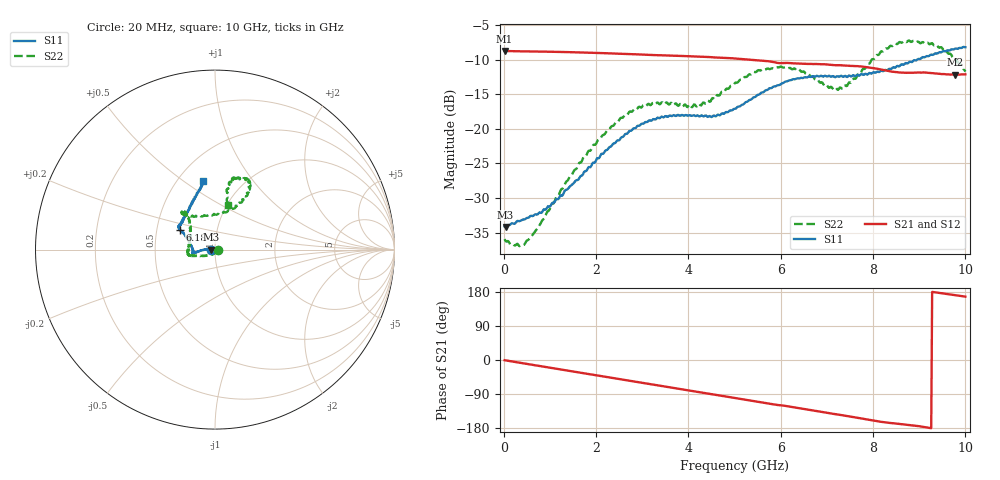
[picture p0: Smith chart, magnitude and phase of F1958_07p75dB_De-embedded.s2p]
! Integrated Device Technology
! Corporate Headquarters
! 6024 Silver Creek Valley Road
! San Jose, CA 95138  USA
! Phone:  1-408-284-8200
! Toll Free:  1-800-223-1366
! Webpage:  http://www.idt.com/
! Timing and RF Division
! 515 Groton Road, Suite 102
! Westford, MA 01886-6024
! Device:  F1958
! Description: 7-bit 0.25 dB Digital Step Attenuator
! Frequency:  0.001 -  6.000 GHz
! Package:  4x4 mm Thin QFN Plastic Package: 24 pin
! Ports:  2 RF, 12 DC
!  Pin  1  = D0
!  Pin  2  = VDD
!  Pin  3  = VMODE
!  Pin  4  = GND
!  Pin  5  = RF1  =  Port 1
!  Pin  6  = GND
!  Pin  7  = GND
!  Pin  8  = GND
!  Pin  9  = GND
!  Pin 10  = GND
!  Pin 11  = GND
!  Pin 12  = GND
!  Pin 13  = GND
!  Pin 14  = RF2  =  Port 2
!  Pin 15  = GND
!  Pin 16  = LE
!  Pin 17  = CLK
!  Pin 18  = DATA
!  Pin 19  = D6
!  Pin 20  = D5
!  Pin 21  = D4
!  Pin 22  = D3
!  Pin 23  = D2
!  Pin 24  = D1
! State:  31
! Atten State:  7.75 dB
! Voltage:  +3.30 Volts
! Current:  0.258 mA
! Data:  The device was measured on a F1958 evaluation board which has
!  individual transmission lines to the RF pins.  Data was collected
!  using a calibrated network analyzer.  The evaluation board was
!  de-embedded using Automatic Fixture Removal (AFR).
!  The reference plane is the edge of the package pin.
! Misc:
!  Action Tracker AT0419
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# GHz S dB R 50
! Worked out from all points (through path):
!   500 points, 20 MHz to 10 GHz, reference 50 ohm
!   highest |S21| = -8.75 dB at 20 MHz (marker M1); lowest = -12.2 dB at 9.78 GHz (marker M2)
!   group delay of S21, straight-line fit = 54.1 ps
!   lowest |S11| = -34.2 dB at 40 MHz (marker M3), VSWR 1.04, Z = 48.1 - j0.0778 ohm
!   |S11| at or under -10 dB: start of sweep to 8.959 GHz
!   |S22| runs from -37.0 to -7.2 dB; largest |S21 - S12| = 0.0011
!   S11 on the Smith chart (normalised r, x): 20 MHz: 0.96, -0.00; 6.18 GHz: 0.66, +0.15; 10 GHz: 0.66, +0.60
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0.02  -34.13 -177.6  -8.75 -0.6  -8.75 -0.5  -35.95 -8.9
0.04  -34.18 -177.6  -8.76 -1.0  -8.76 -0.9  -36.22 -13.5
0.46  -33.07 173.7  -8.82 -9.4  -8.82 -9.4  -36.60 -59.7
0.96  -31.20 175.4  -8.87 -19.5  -8.86 -19.5  -31.91 -105.1
1.7  -26.75 179.8  -8.98 -34.4  -8.98 -34.4  -24.56 -145.7
2.58  -21.18 -173.8  -9.18 -52.0  -9.16 -52.0  -18.40 -163.1
2.92  -19.57 -171.7  -9.26 -58.8  -9.25 -58.9  -16.86 -166.8
3.36  -18.45 -169.5  -9.38 -67.5  -9.38 -67.7  -16.38 -170.4
4.24  -18.23 -173.1  -9.58 -85.0  -9.59 -85.0  -16.43 160.4
4.56  -18.09 -178.7  -9.69 -91.4  -9.70 -91.4  -15.70 146.2
5.02  -17.11 167.3  -9.85 -100.6  -9.86 -100.6  -13.33 132.2
5.54  -15.03 155.9  -10.13 -110.8  -10.14 -110.8  -11.57 129.3
6.18  -13.01 150.6  -10.51 -122.7  -10.52 -122.7  -11.22 131.7
6.68  -12.44 147.8  -10.64 -132.3  -10.66 -132.3  -12.45 126.7
7.06  -12.37 145.1  -10.74 -140.5  -10.75 -140.4  -14.06 108.9
7.3  -12.35 142.7  -10.83 -145.1  -10.83 -145.0  -14.05 91.5
7.9  -12.05 131.8  -11.12 -157.7  -11.12 -157.8  -10.60 62.7
8.34  -11.37 122.2  -11.66 -165.8  -11.67 -165.8  -8.28 59.9
8.74  -10.57 114.5  -11.91 -170.8  -11.92 -170.7  -7.42 64.3
9.24  -9.33 105.0  -11.95 -179.6  -11.96 -179.7  -7.75 74.0
9.78  -8.41 100.4  -12.18 171.3  -12.21 171.3  -9.80 77.8
10  -8.22 99.9  -12.14 167.2  -12.16 167.3  -11.74 73.7
